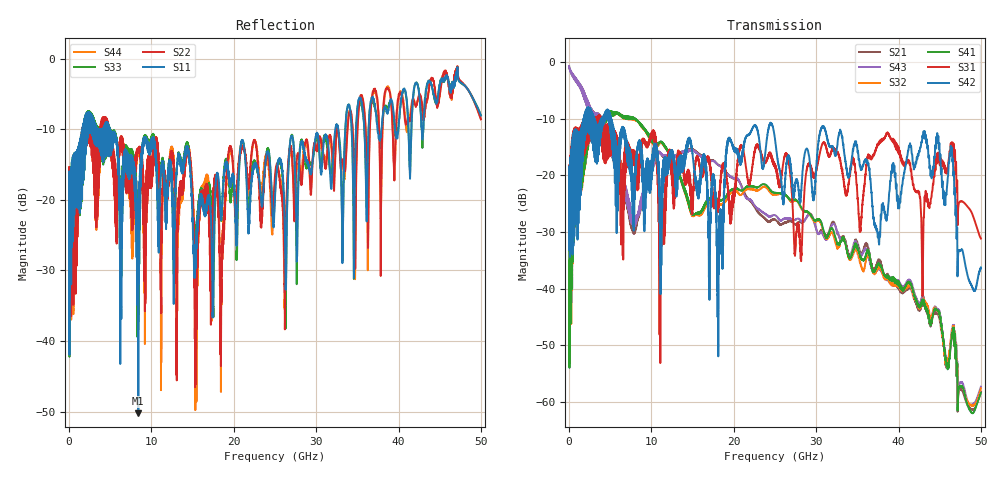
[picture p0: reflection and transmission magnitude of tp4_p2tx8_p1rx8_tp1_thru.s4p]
! 100G CR Analysis
! File: tp4_p2tx8_p1rx8_tp1_thru
! Description: 2m Cu Cable, OSFP, TP1-TP4
! Port Mapping
! Port1 -- P1RX8N
! Port2 -- P2TX8N
! Port3 -- P1RX8P
! Port4 -- P2TX8P
# GHz S MA R 50.00
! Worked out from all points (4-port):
!   5000 points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, 10 MHz to 50 GHz, reference 50 ohm
!   strongest paths, dB at 10 MHz, 12.51 GHz, 25.01 GHz, 37.51 GHz, 50 GHz:
!     S42: -20.6, -15.7, -13.7, -30.7, -36.3
!     S31: -20.5, -17.9, -18.0, -14.7, -31.2
!     S41: -33.3, -17.6, -23.1, -35.8, -58.4
!     S32: -33.3, -17.4, -23.4, -36.5, -57.6
!     S43: -0.7, -16.6, -27.1, -36.6, -57.3
!     S21: -0.7, -16.7, -27.8, -35.2, -58.2
!   lowest |S11| = -50.2 dB at 8.41 GHz (marker M1), VSWR 1.01, Z = 50.2 - j0.204 ohm
!   |S11| at or under -10 dB: start of sweep to 1.658 GHz; 4.913 GHz to 32.33 GHz (27.42 GHz wide, 147 % of centre); 32.69 GHz to 33.54 GHz (850.9 MHz wide, 2.57 % of centre)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
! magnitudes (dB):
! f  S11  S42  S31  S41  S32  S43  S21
! 10 MHz  -18.4  -20.6  -20.5  -33.3  -33.3  -0.7  -0.7
! 2.87 GHz  -10.6  -14.1  -12.7  -10.3  -10.3  -9.2  -9.1
! 8.41 GHz  -50.2  -15.0  -22.4  -10.5  -10.6  -27.2  -27.6
! 15.4 GHz  -27.9  -20.7  -17.4  -26.8  -27.0  -15.9  -15.7
! 37.55 GHz  -10.6  -30.4  -14.3  -35.6  -36.3  -36.4  -35.0
! 43.1 GHz  -7.8  -13.2  -26.8  -43.0  -42.7  -42.6  -43.0
! 50 GHz  -8.0  -36.3  -31.2  -58.4  -57.6  -57.3  -58.2
